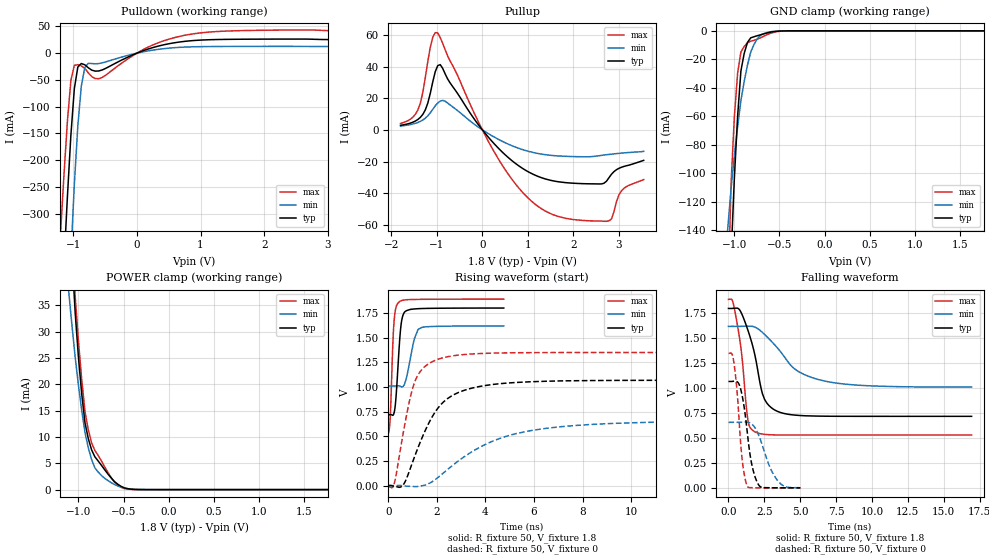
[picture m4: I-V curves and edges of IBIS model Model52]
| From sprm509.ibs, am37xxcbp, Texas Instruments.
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| Model based on original model for BQ18OMAPSMART1HYFBPB_SSBHH
|   Sub model PB_HS10L11_PUPD0_1P8
[model]   Model52
|[Input Load]   PI
|[Output Drive] SC10LB11
|Voltage   1.8V
|Mode   I/O
Model_type   I/O
Polarity   Non-Inverting
Enable   Active-Low
Vinl =  0.63
Vinh =  1.17
Cref =  15pF
Rref =  100.0000M
Vref =  0V
Vmeas =  0.9
C_comp   1.429432p   1.270657p   1.602015p
[Model Spec]
Vinl   0.63   0.567   0.6615
Vinh   1.17   1.053   1.2285
[Temperature Range]   25   125   -40
[Voltage Range]   1.8   1.62   1.89
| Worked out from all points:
|   slope of the pulldown table from 0 to 0.27 V, typ, clamps not added: 24.3 ohm
|   slope of the pullup table from 0 to 0.27 V, typ, clamps not added: 29.7 ohm
|   GND clamp passes 1 mA (typ) near -0.60 V on its own axis
|   POWER clamp passes 1 mA (typ) near -0.56 V on its own axis
|   rising waveform, R_fixture 50, V_fixture 1.8: 20-80 % time 176ps typ, 305ps min, 125ps max; typ from 0.717 V to 1.8 V
|   rising waveform, R_fixture 50, V_fixture 0: 20-80 % time 1.34ns typ, 2.95ns min, 707ps max; typ from 0 V to 1.07 V
|   falling waveform, R_fixture 50, V_fixture 1.8: 20-80 % time 1.04ns typ, 2.54ns min, 610ps max; typ from 1.8 V to 0.718 V
|   falling waveform, R_fixture 50, V_fixture 0: 20-80 % time 613ps typ, 1.03ns min, 440ps max; typ from 1.07 V to 0 V
[POWER_clamp]
-1.8V     362.5mA    191.4mA    412.8mA
-1.109V   56.69mA    37.71mA    60.38mA
-1.073V   44.6mA     31.22mA    47.8mA
-1.036V   33.44mA    25.04mA    36.59mA
-1V       24.98mA    19.72mA    28.06mA
-963.6mV  18.03mA    14.96mA    20.78mA
-927.3mV  12.59mA    10.77mA    14.74mA
-890.9mV  9.653mA    7.899mA    11.31mA
-818.2mV  6.214mA    4.114mA    7.414mA
-636.4mV  2.183mA    1.307mA    2.238mA
-418.2mV  83.85uA    105.2uA    35.14uA
1.764V    -1.228nA   -79.12nA   -1.453nA
[Pulldown]
-1.8V     -1.718A    -2.61A     -1.406A
-1.2V     -527.4mA   -844.5mA   -339.9mA
-1.145V   -396mA     -683.1mA   -229.1mA
-1.091V   -269mA     -526.7mA   -127.5mA
-1.036V   -153.6mA   -378.9mA   -51.17mA
-981.8mV  -66.34mA   -245.6mA   -22.67mA
-927.3mV  -26mA      -136.2mA   -21.54mA
-872.7mV  -19.34mA   -61.98mA   -23.69mA
-763.6mV  -27.2mA    -19.05mA   -36.72mA
-545.5mV  -31.39mA   -18.17mA   -45.46mA
872.7mV   23.46mA    11.88mA    35.92mA
3.545V    25.34mA    12.51mA    41.58mA
[Pullup]
-1.8V     2.903mA    2.423mA    4.112mA
-1.418V   6.595mA    4.711mA    12.64mA
-1.255V   12.69mA    7.42mA     33.23mA
-1.091V   30.4mA     13mA       58.69mA
-981.8mV  40.63mA    17.02mA    61.3mA
-818.2mV  35.38mA    18.12mA    50.59mA
272.7mV   -9.18mA    -4.728mA   -14.55mA
1.255V    -29.75mA   -15.09mA   -48.97mA
2.564V    -34.17mA   -16.31mA   -57.57mA
2.782V    -30.25mA   -15.5mA    -57.48mA
3.055V    -23.63mA   -14.68mA   -38.61mA
3.545V    -19.25mA   -13.56mA   -31.41mA
[GND_clamp]
-1.8V     -2.82A     -1.192A    -3.165A
-1.073V   -235.7mA   -138.4mA   -192.1mA
-1.036V   -159.5mA   -110.8mA   -107.5mA
-1V       -103.8mA   -87.85mA   -60.67mA
-963.6mV  -60mA      -67.28mA   -29.8mA
-927.3mV  -28.21mA   -49.08mA   -14.9mA
-890.9mV  -15.9mA    -35.48mA   -10.99mA
-854.5mV  -8.138mA   -24.07mA   -8.449mA
-818.2mV  -4.924mA   -14.85mA   -7.266mA
-709.1mV  -2.784mA   -3.064mA   -4.883mA
-563.6mV  -570.2uA   -404.5uA   -1.092mA
1.764V    -11.02pA   583.5nA    3.035nA
[Ramp]
dV/dt_f  0.6513625/1.044365n   0.3678568/2.56558n   0.8183097/0.6118918n
dV/dt_r  0.6512914/1.342059n   0.400885/2.971864n   0.8233158/0.7084763n
R_load = 50
[Rising Waveform]
R_fixture = 50
V_fixture = 1.8
V_fixture_min = 1.62
V_fixture_max = 1.89
0s        717.4mV    1.009V     528.5mV
81ps      718.9mV    1.009V     710.6mV
180ps     711.9mV    1.009V     1.41V
234ps     735.3mV    1.009V     1.661V
396ps     1.207V     1.011V     1.849V
522ps     1.629V     1.003V     1.873V
729ps     1.77V      1.078V     1.883V
1.071ns   1.79V      1.488V     1.887V
1.377ns   1.795V     1.603V     1.888V
4.752ns   1.8V       1.618V     1.89V
[Rising Waveform]
R_fixture = 50
V_fixture = 0
V_fixture_min = 0
V_fixture_max = 0
0s        -194.3uV   101.7uV    -10.28mV
234ps     -8.41mV    -225.6uV   11.6mV
612ps     7.284mV    -2.604mV   532.6mV
891ps     164.8mV    -8.102mV   880.9mV
1.125ns   322.6mV    -10.7mV    1.073V
1.701ns   650.3mV    24.24mV    1.242V
2.232ns   838.4mV    120.4mV    1.294V
4.203ns   1.022V     440.3mV    1.342V
6.48ns    1.057V     579.7mV    1.348V
20.3ns    1.067V     655.8mV    1.349V
[Falling Waveform]
R_fixture = 50
V_fixture = 1.8
V_fixture_min = 1.62
V_fixture_max = 1.89
0s        1.8V       1.62V      1.89V
306ps     1.801V     1.62V      1.866V
720ps     1.795V     1.62V      1.552V
1.359ns   1.58V      1.622V     677.3mV
1.809ns   1.354V     1.615V     564.5mV
2.52ns    886.9mV    1.539V     536.9mV
3.708ns   752.5mV    1.351V     530.4mV
4.752ns   728.5mV    1.179V     529.9mV
6.795ns   718.8mV    1.069V     529.8mV
16.94ns   717.6mV    1.011V     529.8mV
[Falling Waveform]
R_fixture = 50
V_fixture = 0
V_fixture_min = 0
V_fixture_max = 0
0s        1.068V     657.4mV    1.349V
243ps     1.068V     657.6mV    1.344V
396ps     1.071V     657.4mV    1.241V
594ps     1.066V     657.4mV    978.7mV
954ps     927.3mV    659.6mV    286.7mV
1.332ns   531.7mV    659.4mV    12.51mV
1.647ns   221mV      637.7mV    1.805mV
2.169ns   17.74mV    506.7mV    211.7uV
3.447ns   351.2uV    69.26mV    5.014uV
5.013ns   54.18uV    1.632mV    543.2nV
